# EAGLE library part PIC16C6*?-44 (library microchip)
MICROCONTROLLER EPROM/ROM-based
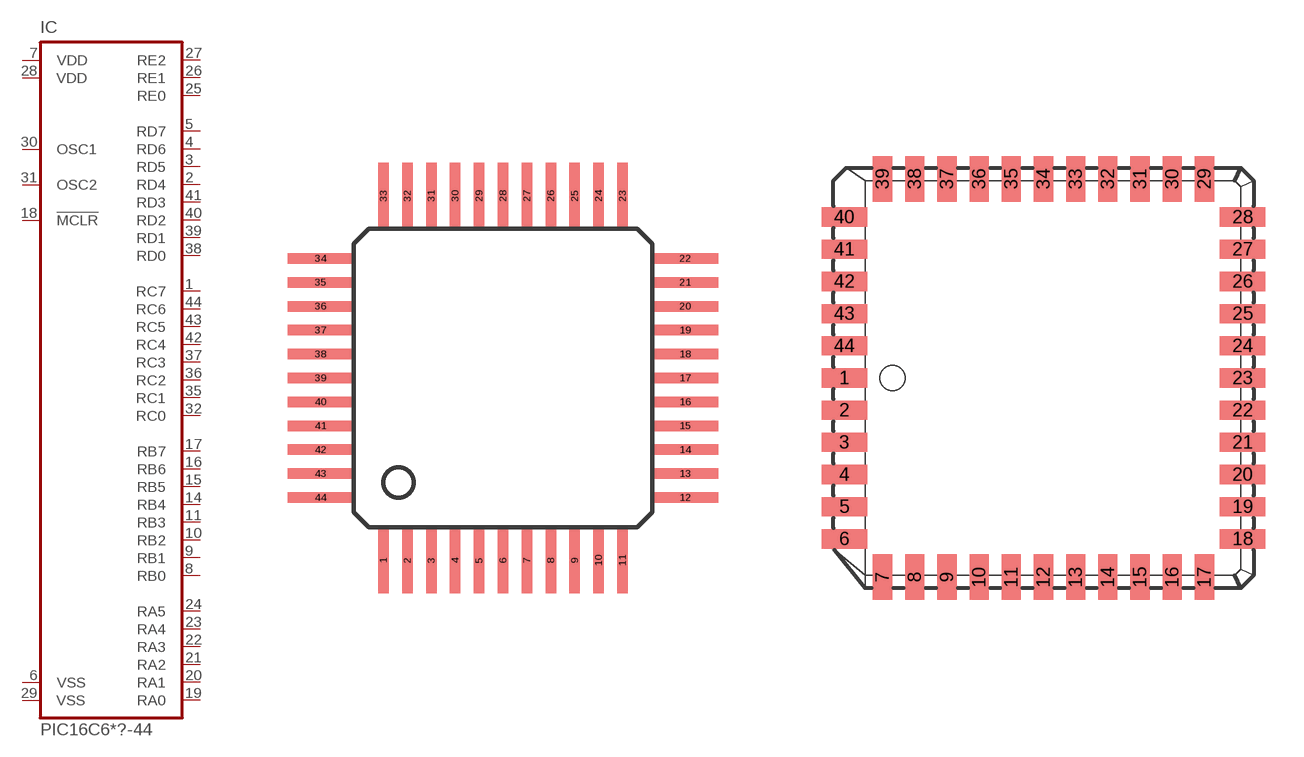
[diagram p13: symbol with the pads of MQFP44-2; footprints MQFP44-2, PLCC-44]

Designator prefix IC

## PIC16C64PQ-44 (MF: MICROCHIP; MPN: PIC16C64A-10I/PT; OC_FARNELL: unknown; OC_NEWARK: 23C4098), PIC16C64APQ-44 (OC_FARNELL: unknown; OC_NEWARK: unknown)  [MQFP44-2]
1  RC7
2  RD4
3  RD5
4  RD6
5  RD7
6  VSS  pwr
7  VDD  pwr
8  RB0
9  RB1
10  RB2
11  RB3
12  NC  nc
13  NC  nc
14  RB4
15  RB5
16  RB6
17  RB7
18  !MCLR  in
19  RA0
20  RA1
21  RA2
22  RA3
23  RA4
24  RA5
25  RE0
26  RE1
27  RE2
28  VDD  pwr
29  VSS  pwr
30  OSC1  in
31  OSC2  out
32  RC0
33  NC  nc
34  NC  nc
35  RC1
36  RC2
37  RC3
38  RD0
39  RD1
40  RD2
41  RD3
42  RC4
43  RC5
44  RC6

## PIC16C64L-44 (MF: MICROCHIP; MPN: PIC16C64A-04/L; OC_FARNELL: 9759646; OC_NEWARK: 96K3813), PIC16C65L-44 (MPN: PIC16C65A-04/L; OC_FARNELL: 9759700; OC_NEWARK: 97K7248)  [PLCC-44]
Pads as for MQFP44-2

## PIC16C64ATQ-44 (MF: MICROCHIP; MPN: PIC16C64A-10I/PT; OC_FARNELL: unknown; OC_NEWARK: 23C4098)  [TQFP44]
Pads as for MQFP44-2

## Footprint MQFP44-2 (pad centres in mm)
Plastic Metric Quad Flat Pack package type PQ
smd 0.35 x 2.2: 1 -4,-6.1; 2 -3.2,-6.1; 3 -2.4,-6.1; 4 -1.6,-6.1; 5 -0.8,-6.1; 6 0,-6.1; 7 0.8,-6.1; 8 1.6,-6.1; 9 2.4,-6.1; 10 3.2,-6.1; 11 4,-6.1; 23 4,6.1; 24 3.2,6.1; 25 2.4,6.1; 26 1.6,6.1; 27 0.8,6.1; 28 0,6.1; 29 -0.8,6.1; 30 -1.6,6.1; 31 -2.4,6.1; 32 -3.2,6.1; 33 -4,6.1
smd 2.2 x 0.35: 12 6.1,-4; 13 6.1,-3.2; 14 6.1,-2.4; 15 6.1,-1.6; 16 6.1,-0.8; 17 6.1,0; 18 6.1,0.8; 19 6.1,1.6; 20 6.1,2.4; 21 6.1,3.2; 22 6.1,4; 34 -6.1,4; 35 -6.1,3.2; 36 -6.1,2.4; 37 -6.1,1.6; 38 -6.1,0.8; 39 -6.1,0; 40 -6.1,-0.8; 41 -6.1,-1.6; 42 -6.1,-2.4; 43 -6.1,-3.2; 44 -6.1,-4

## Footprint PLCC-44 (pad centres in mm)
PLASTIC LEADED CHIP CARRIER square, package type L
smd 1.8 x 0.76: 1 -7.86,0; 2 -7.86,-1.27; 3 -7.86,-2.54; 4 -7.86,-3.81; 5 -7.86,-5.08; 6 -7.86,-6.35; 18 7.86,-6.35; 19 7.86,-5.08; 20 7.86,-3.81; 21 7.86,-2.54; 22 7.86,-1.27; 23 7.86,0; 24 7.86,1.27; 25 7.86,2.54; 26 7.86,3.81; 27 7.86,5.08; 28 7.86,6.35; 40 -7.86,6.35; 41 -7.86,5.08; 42 -7.86,3.81; 43 -7.86,2.54; 44 -7.86,1.27
smd 0.76 x 1.8: 7 -6.35,-7.86; 8 -5.08,-7.86; 9 -3.81,-7.86; 10 -2.54,-7.86; 11 -1.27,-7.86; 12 0,-7.86; 13 1.27,-7.86; 14 2.54,-7.86; 15 3.81,-7.86; 16 5.08,-7.86; 17 6.35,-7.86; 29 6.35,7.86; 30 5.08,7.86; 31 3.81,7.86; 32 2.54,7.86; 33 1.27,7.86; 34 0,7.86; 35 -1.27,7.86; 36 -2.54,7.86; 37 -3.81,7.86; 38 -5.08,7.86; 39 -6.35,7.86

## Footprint TQFP44 (pad centres in mm)
Thin Quad Flat Pack package type TQ
smd 1.5 x 0.5: 1 -5.8,4; 2 -5.8,3.2; 3 -5.8,2.4; 4 -5.8,1.6; 5 -5.8,0.8; 6 -5.8,0; 7 -5.8,-0.8; 8 -5.8,-1.6; 9 -5.8,-2.4; 10 -5.8,-3.2; 11 -5.8,-4; 23 5.8,-4; 24 5.8,-3.2; 25 5.8,-2.4; 26 5.8,-1.6; 27 5.8,-0.8; 28 5.8,0; 29 5.8,0.8; 30 5.8,1.6; 31 5.8,2.4; 32 5.8,3.2; 33 5.8,4
smd 0.5 x 1.5: 12 -4,-5.8; 13 -3.2,-5.8; 14 -2.4,-5.8; 15 -1.6,-5.8; 16 -0.8,-5.8; 17 0,-5.8; 18 0.8,-5.8; 19 1.6,-5.8; 20 2.4,-5.8; 21 3.2,-5.8; 22 4,-5.8; 34 4,5.8; 35 3.2,5.8; 36 2.4,5.8; 37 1.6,5.8; 38 0.8,5.8; 39 0,5.8; 40 -0.8,5.8; 41 -1.6,5.8; 42 -2.4,5.8; 43 -3.2,5.8; 44 -4,5.8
